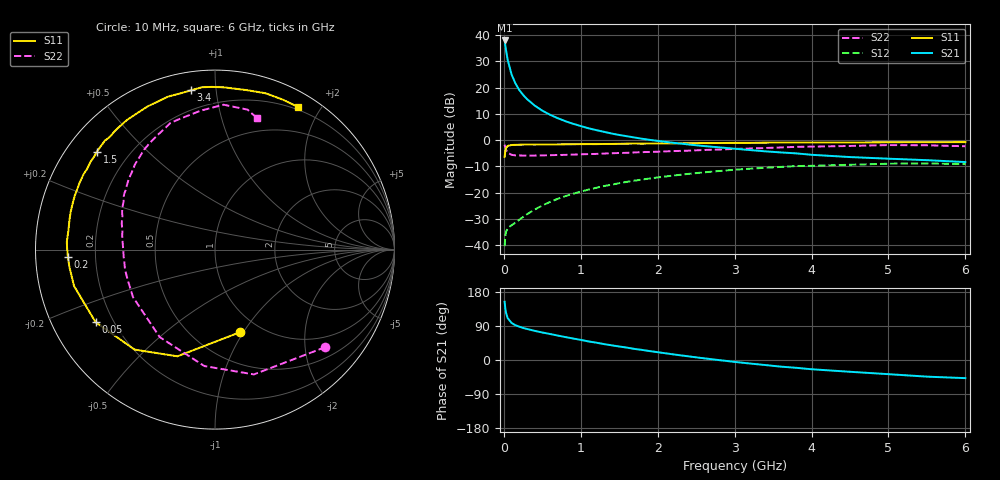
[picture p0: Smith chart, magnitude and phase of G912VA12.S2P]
! SIEMENS Small Signal Semiconductors
! BFG235
! Si NPN RF Bipolar Junction Transistor in SOT223
! VCE = 12 V  IC = 120 mA
! Common Emitter S-Parameters:  July  1994
# GHz  S  MA  R  50
!  f  S11  S21  S12  S22
! GHz  MAG  ANG  MAG  ANG  MAG  ANG  MAG  ANG
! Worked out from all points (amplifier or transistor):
!   40 points, 10 MHz to 6 GHz, reference 50 ohm
!   highest |S21| = 38.0 dB at 10 MHz (marker M1)
!   |S21| within 3 dB of that: start of sweep to 25.19 MHz
!   unconditionally stable (mu >= 1): 475.4 MHz to 1.471 GHz
!   at 200 MHz: K = 0.77, MSG = 24.7 dB, |S12| = -30.3 dB
!   at 1.5 GHz: K = 1.00, MSG = 9.2 dB, |S12| = -16.4 dB
!   at 6 GHz: K = 0.90, MSG = 0.4 dB, |S12| = -9.1 dB
!   S11 on the Smith chart (normalised r, x): 10 MHz: 0.81, -0.97; 50 MHz: 0.13, -0.28; 200 MHz: 0.10, -0.03; 1.5 GHz: 0.09, +0.36; 3.4 GHz: 0.09, +0.86; 6 GHz: 0.17, +1.72
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0.01  0.4809 -73.2  79.46 153.6  0.0096 62.5  0.8202 -41.5
0.02  0.6303 -109.4  63.37 135.2  0.0154 49.4  0.7283 -72.7
0.03  0.7149 -128.8  50.37 123.3  0.0182 40.9  0.6517 -95.2
0.05  0.7784 -148.7  33.86 110.4  0.021 33.5  0.5767 -122.3
0.1  0.8111 -165.5  18 97.9  0.024 35.1  0.528 -149.9
0.15  0.8168 -173.1  12.12 91.8  0.0269 40.2  0.5147 -161.4
0.2  0.8205 -177.0  9.062 87.9  0.0306 45.6  0.5133 -167.6
0.25  0.824 179.5  7.3 84.6  0.0345 49.0  0.5101 -171.7
0.3  0.8267 177.0  6.094 82.0  0.0388 52.1  0.5106 -175.1
0.4  0.8237 172.2  4.582 77.0  0.0477 55.7  0.5109 -179.5
0.5  0.8274 168.6  3.658 72.5  0.0571 57.9  0.5143 177.0
0.6  0.8311 165.5  3.055 68.7  0.0666 58.6  0.5188 173.9
0.7  0.834 161.7  2.631 64.4  0.0766 59.0  0.5232 171.2
0.9  0.8382 156.3  2.058 56.7  0.0955 57.6  0.532 166.6
1.1  0.8443 149.9  1.689 49.0  0.1147 55.3  0.5444 162.1
1.5  0.8549 140.3  1.258 35.6  0.152 49.3  0.5709 154.0
2.2  0.8729 124.2  0.894 14.9  0.2122 37.2  0.6211 140.7
3.2  0.8914 102.7  0.649 -9.3  0.2866 17.9  0.6955 121.7
3.4  0.8975 98.5  0.614 -13.3  0.2985 13.9  0.7113 117.3
4.5  0.9059 78.8  0.478 -31.1  0.3407 -7.2  0.7779 96.0
5.5  0.9169 65.6  0.417 -43.9  0.3616 -25.7  0.8006 76.9
6  0.9192 59.9  0.384 -47.9  0.3511 -32.5  0.7679 72.1
